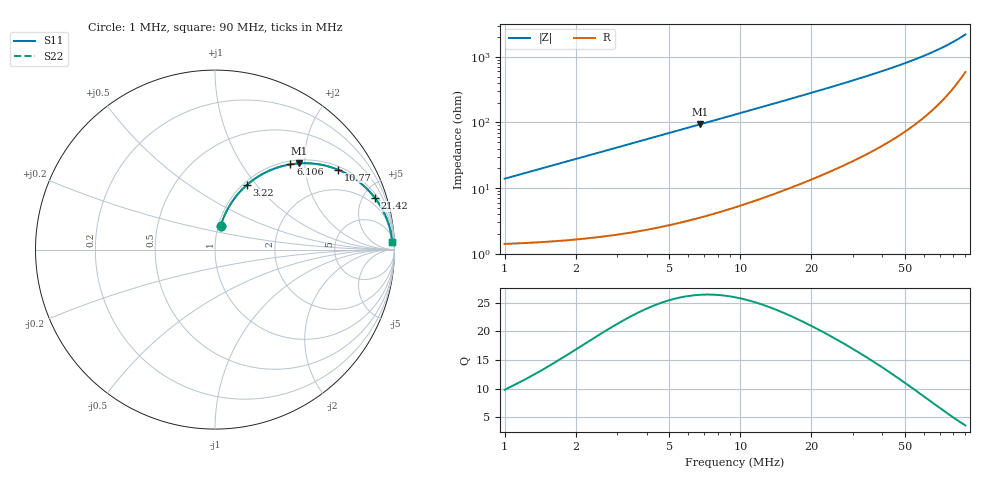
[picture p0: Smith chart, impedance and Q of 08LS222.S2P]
! Coilcraft 0805LS-222 Chip Inductor
! 18 September 2002
# MHZ S MA R 50
!Freq  MagS11  AngS11  MagS21  AngS21  MagS12  AngS12  MagS22  AngS22
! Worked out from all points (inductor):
!   402 points, 1 MHz to 90 MHz, reference 50 ohm
!   read as one part in series: L = 2.2 uH near 1.444 MHz
!   highest Q = 26.4 at 6.772 MHz (marker M1), where L = 2.2 uH
!   S11 on the Smith chart (normalised r, x): 1 MHz: 1.03, +0.28; 3.22 MHz: 1.04, +0.89; 6.106 MHz: 1.06, +1.69; 10.77 MHz: 1.12, +2.99; 21.42 MHz: 1.30, +6.07; 90 MHz: 13, +42
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1  0.1358 76.4  0.9771 -7.8  0.9771 -7.8  0.1358 76.4
1.222  0.1648 75.6  0.9723 -9.5  0.9723 -9.5  0.1648 75.6
1.666  0.2217 73.4  0.9603 -12.8  0.9603 -12.8  0.2217 73.4
2.11  0.2762 70.7  0.9454 -16.0  0.9454 -16.0  0.2762 70.7
2.554  0.3281 67.9  0.928 -19.1  0.928 -19.1  0.3281 67.9
3.22  0.4004 63.8  0.8983 -23.6  0.8983 -23.6  0.4004 63.8
3.886  0.4656 59.9  0.8656 -27.7  0.8656 -27.7  0.4656 59.9
4.552  0.5238 56.1  0.8311 -31.6  0.8311 -31.6  0.5238 56.1
6.106  0.6341 48.5  0.7495 -39.3  0.7495 -39.3  0.6341 48.5
6.772  0.6718 45.7  0.7157 -42.2  0.7157 -42.2  0.6718 45.7
8.77  0.7587 38.5  0.6231 -49.3  0.6231 -49.3  0.7587 38.5
10.768  0.817 33.0  0.5454 -54.7  0.5454 -54.7  0.817 33.0
13.21  0.8642 27.9  0.4687 -59.7  0.4687 -59.7  0.8642 27.9
15.874  0.8976 23.8  0.4034 -63.7  0.4034 -63.7  0.8976 23.8
18.538  0.9198 20.6  0.3522 -66.8  0.3522 -66.8  0.9198 20.6
21.424  0.9363 17.9  0.3082 -69.3  0.3082 -69.3  0.9363 17.9
25.642  0.9521 15.0  0.2588 -71.9  0.2588 -71.9  0.9521 15.0
30.748  0.9639 12.4  0.2149 -74.2  0.2149 -74.2  0.9639 12.4
45.622  0.9793 7.9  0.1374 -77.4  0.1374 -77.4  0.9793 7.9
60.496  0.9847 5.4  0.09403 -78.0  0.09403 -78.0  0.9847 5.4
75.37  0.9867 3.7  0.06543 -76.4  0.06543 -76.4  0.9867 3.7
90  0.987 2.5  0.04507 -72.0  0.04507 -72.0  0.987 2.5
